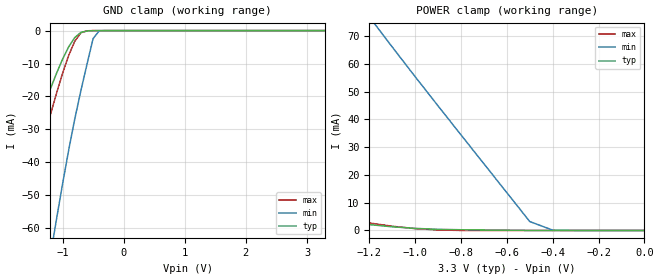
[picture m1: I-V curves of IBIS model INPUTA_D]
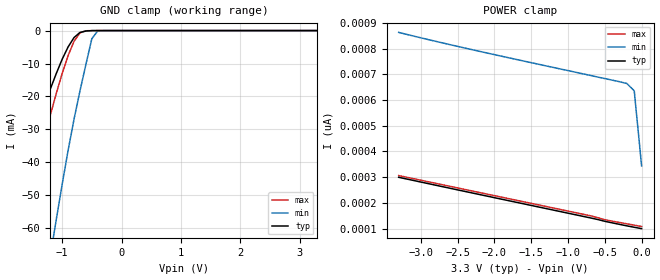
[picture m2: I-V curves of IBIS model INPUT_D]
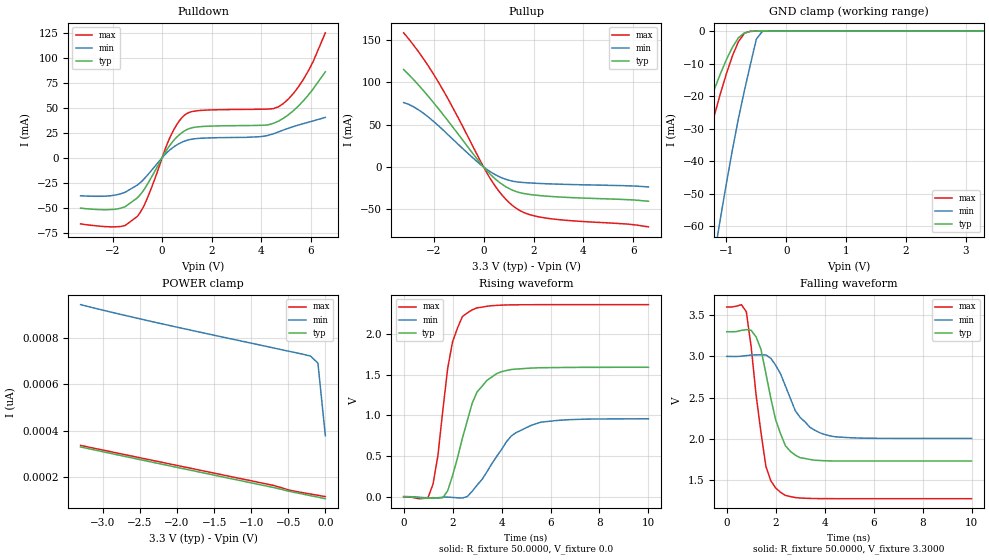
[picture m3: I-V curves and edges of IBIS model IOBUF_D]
| Integrated Devices Technolgy, Inc.
| IBIS MODEL OF 82v2048 / 82v2058
| PQFP_144_DA Package
[Ibis Ver]   3.2
[File Name]   2058pqfp.ibs
[File Rev]   1.0
[Date]   09/14/2005 zsy
[Source]   Integrated Devices Technolgy, Inc.
[Notes]   11/16/2001 zym
   1. Temperatures: typ=25C, min=85C, max=-40C.
   09/14/2005 zsy
   1. C_comp is Updated.
   2. OUTPUTA is removed.
   3. IBIS models are validated with HSPice model.
[Disclaimer] Integrated Device Technology, Inc. ("IDT") hereby grants the
   user of this IBIS model a non-exclusive, nontransferable
   license to use this IBIS model under the following terms. The
   user is granted this license only to use the IBIS model and is
   not granted rights to sell, copy (except as needed to run the
   IBIS model), rent, lease or sub-license the IBIS model in
   whole or in part, or in modified form to anyone. The User may
   modify the IBIS model to suit its specific applications, but
   rights to derivative works and such modifications shall belong
   to IDT. This IBIS model is provided on an AS IS" basis and IDT
   makes absolutely no warranty with respect to the information
   contained herein. IDT DISCLAIMS AND CUSTOMER WAIVES ALL
   WARRANTIES, EXPRESS AND IMPLIED, INCLUDING WARRANTIES OF
   MERCHANTABILITY AND FITNESS FOR A PARTICULAR PURPOSE. THE
   ENTIRE RISK AS TO QUALITY AND PERFORMANCE IS WITH THE USER
   ACCORDINGLY, IN NO EVENT SHALL IDT BE LIABLE FOR ANY DIRECT OR
   INDIRECT DAMAGES, WHETHER IN CONTRACT OR TORT, INCLUDING ANY
   LOST PROFITS OR OTHER INCIDENTAL, CONSEQUENTIAL, EXEMPLARY, OR
   PUNITIVE DAMAGES ARISING OUT OF THE USE OR APPLICATION OF THE
   IBIS model. Further, IDT reserves the right to make changes
   without notice to any product herein to improve reliability,
   function, or design. IDT does not convey any license under
   patent rights or any other intellectual property rights,
   including those of third parties. IDT is not obligated to
   provide maintenance or support for the licensed IBIS model.
[Copyright]   Copyright 2001, Integrated Devices Technolgy, Inc. all rights
   reserved
|   Component 82v2048p
[Component]   2048_58p
[Manufacturer]   Integrated Devices Technolgy, Inc.
[Package]
| variable   typ   min   max
R_pkg   117.6m   111.5m   123.7m
L_pkg   6.90nH   5.74nH   8.05nH
C_pkg   1.23pF   1.221pF   1.243pF
|   Pin List ( 144 PQFP )
[PIN]   signal_name   Model_name   R_pin   L_pin   C_pin
   1   TD7/TDP7   INPUT_D
   2   TCLK7   INPUT_D
   3   LOS6   OUTPUT_D
   4   CV6/RDN6   OUTTRI2_D
   5   RD6/RDP6   OUTTRI2_D
   6   RCLK6   OUTTRI2_D
   7   BPVI6/TDN6   INPUT_D
   8   TD6/TDP6   INPUT_D
   9   TCLK6   INPUT_D
   10   MCLK   INPUT_D
   11   MODE2   INPUT_D
   12   MC4/A4   INPUT_D
   13   MC3/A3   INPUT_D
   14   MC2/A2   INPUT_D
   15   MC1/A1   INPUT_D
   16   MC0/A0   INPUT_D
   17   VDDIO   POWER
   18   GNDIO   GND
   19   VDDD   POWER
   20   GNDD   GND
   21   LOP0/D0/AD0   IOBUF_D
   22   LOP1/D1/AD1   IOBUF_D
   23   LOP2/D2/AD2   IOBUF_D
   24   LOP3/D3/AD3   IOBUF_D
   25   LOP4/D4/AD4   IOBUF_D
   26   LOP5/D5/AD5   IOBUF_D
   27   LOP6/D6/AD6   IOBUF_D
   28   LOP7/D7/AD7   IOBUF_D
   29   TCLK1   INPUT_D
   30   TD1/TDP1   INPUT_D
   31   BPVI1/TDN1   INPUT_D
   32   RCLK1   OUTTRI2_D
   33   RD1/RDP1   OUTTRI2_D
   34   CV1/RDN1   OUTTRI2_D
   35   LOS1   OUTPUT_D
   36   TCLK0   INPUT_D
   37   TD0/TDP0   INPUT_D
   38   BPVI0/TDN0   INPUT_D
   39   RCLK0   OUTTRI2_D
   40   RD0/RDP0   OUTTRI2_D
   41   CV0/RDN0   OUTTRI2_D
   42   LOS0   OUTPUT_D
   43   MODE1   INPUT_D
   44   VDDT0   POWER
   45   TTIP0   NC
   46   TRING0   NC
   47   GNDT0   GND
   48   RTIP0   INPUTA_D
   49   RRING0   INPUTA_D
   50   GNDT1   GND
   51   TRING1   NC
   52   TTIP1   NC
   53   VDDT1   POWER
   54   RRING1   INPUTA_D
   55   RTIP1   INPUTA_D
   56   VDDT2   POWER
   57   TTIP2   NC
   58   TRING2   NC
   59   GNDT2   GND
   60   RTIP2   INPUTA_D
   61   RRING2   INPUTA_D
   62   GNDT3   GND
   63   TRING3   NC
   64   TTIP3   NC
   65   VDDT3   POWER
   66   RRING3   INPUTA_D
   67   RTIP3   INPUTA_D
   68   LOS3   OUTPUT_D
   69   CV3/RDN3   OUTTRI2_D
   70   RD3/RDP3   OUTTRI2_D
   71   RCLK3   OUTTRI2_D
   72   BPVI3/TDN3   INPUT_D
   73   TD3/TDP3   INPUT_D
   74   TCLK3   INPUT_D
   75   LOS2   OUTPUT_D
   76   CV2/RDN2   OUTTRI2_D
   77   RD2/RDP2   OUTTRI2_D
   78   RCLK2   OUTTRI2_D
   79   BPVI2/TDN2   INPUT_D
   80   TD2/TDP2   INPUT_D
   81   TCLK2   INPUT_D
   82   INT_   OUTDRN_D
   83   SDO/RDY/ACK_   OUTTRI_D
   84   TS0/SDI/WR_/DS_   INPUT_D
   85   TS1/RD_/R/W_   INPUT_D
   86   TS2/SULK/ALE/AS_   INPUT_D
   87   CS_/JAS   INPUT_D
   88   MODE0/CODE   INPUT_D
   89   GNDA   GND
   90   VDDA   POWER
   91   GNDIO   GND
   92   VDDIO   POWER
   95   TRST_   INPUT_D
   96   TMS   INPUT_D
   97   TCK   INPUT_D
   98   TDO   OUTTRI_D
   99   TDI   INPUT_D
   100   TCLK5   INPUT_D
   101   TD5/TDP5   INPUT_D
   102   BPVI5/TDN5   INPUT_D
   103   RCLK5   OUTTRI2_D
   104   RD5/RDP5   OUTTRI2_D
   105   CV5/RDN5   OUTTRI2_D
   106   LOS5   OUTPUT_D
   107   TCLK4   INPUT_D
   108   TD4/TDP4   INPUT_D
   109   BPVI4/TDN4   INPUT_D
   110   RCLK4   OUTTRI2_D
   111   RD4/RDP4   OUTTRI2_D
   112   CV4/RDN4   OUTTRI2_D
   113   LOS4   OUTPUT_D
   114   OE   INPUT_D
   115   CLKE   INPUT_D
   116   VDDT4   POWER
   117   TTIP4   NC
   118   TRING4   NC
   119   GND4   GND
   120   RTIP4   INPUTA_D
   121   RRING4   INPUTA_D
   122   GNDT5   GND
   123   TRING5   NC
   124   TTIP5   NC
   125   VDDT5   POWER
   126   RRING5   INPUTA_D
   127   RTIP5   INPUTA_D
   128   VDDT6   POWER
   129   TTIP6   NC
   130   TRING6   NC
   131   GNDT6   GND
   132   RTIP6   INPUTA_D
   133   RRING6   INPUTA_D
   134   GNDT7   GND
   135   TRING7   NC
   136   TTIP7   NC
   137   VDDT7   POWER
   138   RRING7   INPUTA_D
   139   RTIP7   INPUTA_D
   140   LOS7   OUTPUT_D
   141   CV7/RDN7   OUTTRI2_D
   142   RD7/RDP7   OUTTRI2_D
   143   RCLK7   OUTTRI2_D
   144   BPVII7/TDN7   INPUT_D
| Models and submodels in the file (7): INPUTA_D (Input), INPUT_D (Input), IOBUF_D (I/O), OUTDRN_D (Open_drain), OUTPUT_D (Output), OUTTRI2_D (3-state), OUTTRI_D (3-state)
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|   Model INPUTA_D
[Model]   INPUTA_D
Model_type   Input
Polarity   Non-Inverting
Vinl =   0.8000V
Vinh =   2.0000V
C_comp   2.6600pF   2.5500pF   2.7500pF
[Temperature Range]   25.0000   85.0000   -40.0000
[Voltage Range]   3.3000V   3.0000V   3.6000V
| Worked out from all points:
|   GND clamp passes 1 mA (typ) near -0.73 V on its own axis
|   POWER clamp passes 1 mA (typ) near -1.04 V on its own axis
[GND_clamp]
|Voltage   I(typ)   I(min)   I(max)
-3.3V     -137.1mA   -322.6mA   -175.3mA
-2V       -62.29mA   -163.4mA   -83.75mA
-1.9V     -56.42mA   -151.2mA   -76.37mA
-1.7V     -44.81mA   -127mA     -61.58mA
-1.2V     -17.78mA   -68.55mA   -25.7mA
-1.1V     -13.07mA   -57.42mA   -19.14mA
-900mV    -4.968mA   -36.37mA   -7.604mA
-800mV    -2.123mA   -26.9mA    -3.261mA
-700mV    -567.3uA   -18.29mA   -686.2uA
-500mV    -20.03uA   -2.454mA   -2.991uA
-400mV    -558.3nA   -104.1uA   -83.1nA
3.3V      99.56pA    4.972uA    90.58pA
[POWER_clamp]
|Voltage   I(typ)   I(min)   I(max)
-3.3V     40mA       321.7mA    54.47mA
-2.6V     24.96mA    237.9mA    34.72mA
-2.3V     18.92mA    202.4mA    26.52mA
-2V       13.31mA    167.4mA    18.76mA
-1.6V     6.825mA    121.4mA    9.569mA
-1.4V     4.195mA    98.97mA    5.754mA
-1.2V     2.116mA    76.9mA     2.7mA
-1.1V     1.33mA     66.06mA    1.535mA
-900mV    413.2uA    44.84mA    182uA
-500mV    19.48uA    3.21mA     5.772nA
-400mV    397.5nA    126.9uA    170.8pA
0V        99.59pA    343.8pA    108pA
|   Model INPUT_D
[Model]   INPUT_D
Model_type   Input
Polarity   Non-Inverting
Vinl =   0.8000V
Vinh =   2.0000V
C_comp   2.6600pF   2.5500pF   2.7500pF
[Temperature Range]   25.0000   85.0000   -40.0000
[Voltage Range]   3.3000V   3.0000V   3.6000V
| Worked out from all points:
|   GND clamp passes 1 mA (typ) near -0.73 V on its own axis
[GND_clamp]
|Voltage   I(typ)   I(min)   I(max)
-3.3V     -137.1mA   -322.6mA   -175.3mA
-2V       -62.29mA   -163.4mA   -83.75mA
-1.9V     -56.42mA   -151.2mA   -76.37mA
-1.7V     -44.81mA   -127mA     -61.58mA
-1.2V     -17.78mA   -68.55mA   -25.7mA
-1.1V     -13.07mA   -57.42mA   -19.14mA
-900mV    -4.968mA   -36.37mA   -7.604mA
-800mV    -2.123mA   -26.9mA    -3.261mA
-700mV    -567.3uA   -18.29mA   -686.2uA
-500mV    -20.03uA   -2.454mA   -2.991uA
-400mV    -558.3nA   -104.1uA   -83.11nA
3.3V      99.56pA    671pA      92.43pA
[POWER_clamp]
|Voltage   I(typ)   I(min)   I(max)
-3.3V     299.3pA    862.7pA    306pA
-2.4V     244.4pA    801.8pA    252pA
-700mV    141.7pA    695.6pA    150pA
-500mV    128.2pA    683.2pA    134.4pA
-200mV    110.5pA    663.9pA    118.4pA
-100mV    105pA      635.5pA    113.2pA
0V        99.59pA    343.8pA    108pA
|   Model IOBUF_D
[Model]   IOBUF_D
Model_type   I/O
Polarity   Non-Inverting
Enable   Active-Low
Vinl =   0.8000V
Vinh =   2.0000V
Vmeas =   1.65V
C_comp   2.6600pF   2.5500pF   2.7500pF
[Temperature Range]   25.0000   85.0000   -40.0000
[Voltage Range]   3.3000V   3.0000V   3.6000V
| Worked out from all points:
|   slope of the pulldown table from 0 to 0.495 V, typ, clamps not added: 27.4 ohm
|   slope of the pullup table from 0 to 0.495 V, typ, clamps not added: 33.3 ohm
|   GND clamp passes 1 mA (typ) near -0.73 V on its own axis
|   rising waveform, R_fixture 50.0000, V_fixture 0.0: 20-80 % time 924ps typ, 1.35ns min, 609ps max; typ from 0 V to 1.59 V
|   falling waveform, R_fixture 50.0000, V_fixture 3.3000: 20-80 % time 754ps typ, 1.03ns min, 575ps max; typ from 3.3 V to 1.73 V
[Pulldown]
|Voltage   I(typ)   I(min)   I(max)
-3.3V     -50.6mA    -38.2mA    -66.3mA
-1.7V     -50.82mA   -36.4mA    -69.02mA
-1V       -40.22mA   -27.41mA   -58.83mA
-600mV    -26.75mA   -17.69mA   -40.63mA
400mV     15.28mA    9.501mA    24.65mA
700mV     23.09mA    14.29mA    37.06mA
1V        28.14mA    17.37mA    44.25mA
4.2V      32.68mA    21.86mA    48.65mA
4.9V      39.41mA    27.66mA    54.22mA
5.7V      56.65mA    34.04mA    77.97mA
6.1V      68.64mA    36.79mA    95.93mA
6.6V      86.05mA    40.32mA    125.1mA
[Pullup]
|Voltage   I(typ)   I(min)   I(max)
-3.2V     115.2mA    76.13mA    158.6mA
-2.6V     96.71mA    67.48mA    136.1mA
-1.8V     68.68mA    48.58mA    99.92mA
-1V       38.15mA    26.3mA     57.23mA
100mV     -3.385mA   -2.22mA    -5.351mA
600mV     -17.41mA   -11.11mA   -28.06mA
900mV     -23.53mA   -14.7mA    -38.48mA
1.2V      -27.95mA   -16.99mA   -46.54mA
1.7V      -31.86mA   -18.61mA   -54.89mA
2.5V      -34.45mA   -19.82mA   -60.41mA
5.7V      -38.6mA    -22.2mA    -67.39mA
6.6V      -40.5mA    -23.6mA    -70.8mA
[GND_clamp]
|Voltage   I(typ)   I(min)   I(max)
-3.3V     -137.1mA   -322.6mA   -175.3mA
-2V       -62.29mA   -163.4mA   -83.75mA
-1.9V     -56.42mA   -151.2mA   -76.37mA
-1.7V     -44.82mA   -127mA     -61.58mA
-1.2V     -17.78mA   -68.52mA   -25.71mA
-1.1V     -13.08mA   -57.44mA   -19.15mA
-900mV    -4.991mA   -36.43mA   -7.626mA
-800mV    -2.068mA   -26.9mA    -3.261mA
-700mV    -567.3uA   -18.29mA   -686.2uA
-500mV    -20.03uA   -2.454mA   -2.991uA
-400mV    -558.3nA   -104.1uA   -83.12nA
3.3V      108pA      728.4pA    100.3pA
[POWER_clamp]
|Voltage   I(typ)   I(min)   I(max)
-3.3V     330.2pA    941.5pA    336.8pA
-2.3V     262.6pA    866.1pA    270.7pA
-700mV    156.1pA    755.6pA    165pA
-500mV    140.6pA    741.9pA    146pA
-200mV    121pA      720.7pA    128pA
-100mV    114.7pA    690.4pA    122.5pA
0V        108pA      378.7pA    117pA
[Ramp]
| variable   typ   min   max
dV/dt_r   0.9564/0.9707n   0.5757/1.4116n   1.4190/0.5942n
dV/dt_f   0.9420/0.7459n   0.5970/1.0203n   1.3962/0.4926n
R_load =   50.0000
[Rising Waveform]
R_fixture=   50.0000
V_fixture=   0.0
V_fixture_min=  0.0
V_fixture_max=  0.0
|time   V(typ)   V(min)   V(max)
0s        0V         0V         0V
1ns       -18.22mV   -13.26mV   -9.747mV
1.2ns     -11.95mV   -15.93mV   155.1mV
1.4ns     -18.92mV   -12.91mV   507.1mV
1.8ns     73.29mV    -5.505mV   1.583V
2.4ns     719.6mV    -16.72mV   2.219V
3ns       1.291V     142.1mV    2.326V
4ns       1.54V      580.9mV    2.36V
5.6ns     1.588V     916.9mV    2.365V
10ns      1.594V     959.5mV    2.365V
[Falling Waveform]
R_fixture=   50.0000
V_fixture=   3.3000
V_fixture_min=  3.0000
V_fixture_max=  3.6000
|time   V(typ)   V(min)   V(max)
0s        3.3V       3V         3.6V
800ps     3.325V     3.01V      3.542V
1ns       3.317V     3.016V     3.111V
1.2ns     3.236V     3.019V     2.53V
1.6ns     2.794V     3.018V     1.665V
2ns       2.23V      2.893V     1.403V
2.2ns     2.059V     2.788V     1.349V
3ns       1.77V      2.259V     1.281V
4ns       1.734V     2.053V     1.274V
10ns      1.73V      2.005V     1.273V
